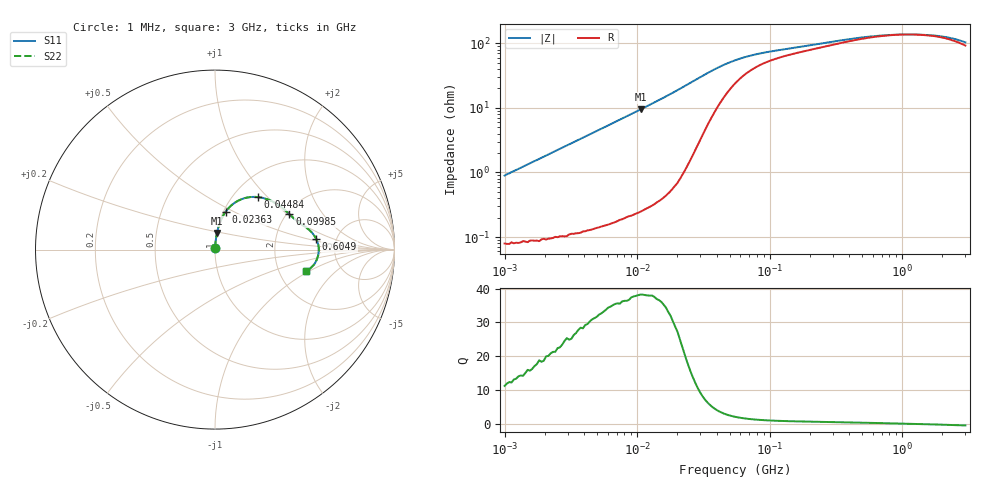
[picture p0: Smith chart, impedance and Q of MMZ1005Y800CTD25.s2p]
! S-Parameter Data Generated by TDK Corporation
! Copyright(C) 2025 TDK Corporation.
! All Rights Reserved.
! TDK P/N: MMZ1005Y800CTD25 (Chip Bead)
! Property: |Z|=80ohm at 100MHz
! Size(LxWxT): 1x0.5x0.5mm
! Model Type: s2p (Touchstone File Format Version 1.0)
! Frequency: DC=Yes Start=1MHz Stop=3000MHz 202points Log-sweep
! Model Generated on Feb. 6, 2025
! Terms and conditions regarding TDK Simulation Models:
! 1)This simulation model is being provided solely for informational
!  purposes. Please refer to the specifications of the products in
!  terms of detailed characteristics of such products.
! 2)In no event shall TDK Corporation of any of its subsidiaries be
!  liable for any loss or damage arising, directly or indirectly,
!  from any information contained in this simulation model, including,
!  but not limited to loss or damages arising from any inaccuracies,
!  omissions or errors in connection with such information.
! 3)Any and all copyrights on this simulation model are owned by
!  TDK Corporation.  Duplication or redistribution of this simulation
!  model without prior written permission from TDK Corporation
!  is prohibited.
! 4)This simulation model is subject to any modification or change
!  without any prior notice.
! 5)Neither TDK Corporation nor any of its subsidiaries shall make any
!  warranty, express or implied, including but not limited to the
!  correctness, implied warranties of merchantability and fitness for
!  a particular purpose with respect to this simulation models.
! 6)The use of this simulation model shall be deemed to have consented
!  to the terms and conditions hereof.
! Port Assignments:
!  1 ---@@@--- 2
! Applicable Conditions:
!  Temperature = 25 degC
!  DC Bias Current = 0 A
!  Small Signal Operation
# Hz S MA R 50
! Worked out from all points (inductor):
!   201 points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, 1 MHz to 3 GHz, reference 50 ohm
!   read as one part in series: L = 142 nH near 1.041 MHz
!   highest Q = 38.1 at 10.61 MHz (marker M1), where L = 142 nH
!   self-resonance near 1.112 GHz
!   S11 on the Smith chart (normalised r, x): 1 MHz: 1.00, +0.02; 23.63 MHz: 1.02, +0.45; 44.84 MHz: 1.29, +0.88; 99.85 MHz: 2.07, +1.03; 604.9 MHz: 3.50, +0.61; 3 GHz: 2.85, -0.94
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1000000  0.008932 84.4  0.9992 -0.5  0.9992 -0.5  0.008932 84.4
3900413  0.03452 86.0  0.9982 -2.0  0.9982 -2.0  0.03452 86.0
6831390  0.06032 84.9  0.9965 -3.5  0.9965 -3.5  0.06032 84.9
1.061086e7  0.09399 83.1  0.9931 -5.4  0.9931 -5.4  0.09399 83.1
1.461624e7  0.1306 80.9  0.9879 -7.5  0.9879 -7.5  0.1306 80.9
1.934349e7  0.1758 77.9  0.9784 -10.1  0.9784 -10.1  0.1758 77.9
2.362996e7  0.2183 74.4  0.9643 -12.6  0.9643 -12.6  0.2183 74.4
2.773354e7  0.2584 70.2  0.9444 -14.9  0.9444 -14.9  0.2584 70.2
3.387922e7  0.3116 63.1  0.9029 -17.9  0.9029 -17.9  0.3116 63.1
3.820236e7  0.3422 58.1  0.869 -19.5  0.869 -19.5  0.3422 58.1
4.483659e7  0.377 50.9  0.8165 -21.0  0.8165 -21.0  0.377 50.9
5.477226e7  0.4096 42.5  0.7506 -21.6  0.7506 -21.6  0.4096 42.5
6.964249e7  0.435 34.1  0.6845 -20.9  0.6845 -20.9  0.435 34.1
9.984923e7  0.4592 25.4  0.6176 -18.6  0.6176 -18.6  0.4592 25.4
2.136344e8  0.5052 15.9  0.5325 -15.1  0.5325 -15.1  0.5052 15.9
3.741707e8  0.5436 10.7  0.4766 -12.2  0.4766 -12.2  0.5436 10.7
6.049187e8  0.5671 6.0  0.4401 -7.8  0.4401 -7.8  0.5671 6.0
8.005644e8  0.575 3.3  0.4272 -4.4  0.4272 -4.4  0.575 3.3
1.243477e9  0.5782 -1.1  0.4221 1.6  0.4221 1.6  0.5782 -1.1
1.782824e9  0.5714 -5.2  0.4341 6.9  0.4341 6.9  0.5714 -5.2
2.359433e9  0.554 -9.2  0.4619 11.1  0.4619 11.1  0.554 -9.2
3e9  0.5233 -13.2  0.5048 13.7  0.5048 13.7  0.5233 -13.2
